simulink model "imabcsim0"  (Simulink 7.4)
settings: Solver=ode45  StartTime=0.0  StopTime=8  RelTol=1e-3
InitFcn:
  | imparamsim0
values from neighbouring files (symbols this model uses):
  Bm = 0.10    (= 0.1)    [IMabc2.m]    (also in imabcparam.m = 0.01; IMabcrun0.m = 0.01; IMabcrun1.m = 0.001; IMcur0.m = 1e-06)
  D = str2num(get(h,'string'))    [acttrcalc1.m]
  gam = 2*pi/3    (= 2.09439510239)    [IMabc2.m]    (also in IMabcf0.m; IMabcf1.m; imabcparam.m; IMabcrun0.m)
  J = 0.02    [imabcparam.m]    (also in IMabcrun0.m; IMabcrun1.m; imdefSIvec1.m = 0.03)
  Lm1 = 2/3*Lm    [IMabcf0.m]    (also in IMabcf1.m; imabcparam.m = 0.0564666666667; IMabcrun0.m = 0.0564666666667; IMabcrun1.m = 0.0564666666667)
  Lr = Lrl+Lm    (= 4.6)    [IMabc2.m]    (also in IMabcf0.m = Lrl+Lm1; IMabcf1.m = Lrl+Lm1; imabcparam.m = 0.0589666666667; IMcur0.m)
  Ls = Lsl+Lm    (= 4.6)    [IMabc2.m]    (also in IMabcf0.m = Lsl+Lm1; IMabcf1.m = Lsl+Lm1; imabcparam.m = 0.0589666666667; IMcur0.m)
  nsync = 120*freq0/p    (= 1800)    [imabcparam.m]
  p = cos(beta-alpha)    [abcRwdg.m]    (also in alternator.m = 0:pi/20:2*pi; altwdgs.m = 0:pi/20:2*pi; brushlessdcB.m = 0:pi/100:2*pi; brushlessdcnew.m = 0:pi/100:2*pi)
  Rr = input('Rotor resistance)[default = 2] =')    [Actac.m]    (also in im1phase.m = 0.3; im3d.m = eval(get(hRr,'String')); IMabc2.m = 0.02; imabcparam.m = 0.408)
  Rs = eval(get(hRs,'String'))    [im3d.m]    (also in IMabc2.m = 0.01; imabcparam.m = 0.531; IMabcrun0.m = 0.531; IMabcrun1.m = 0.531)
  Vm = Vll*sqrt(2/3)    [imabcparam.m]
  wo = 2*pi*freq0    [calc0.m]    (also in IMabc2.m = 376.991118431; imabcparam.m = 376.991118431; IMabcrun0.m = 376.991118431; IMabcrun1.m = 376.991118431)
undefined symbols (not defined in the file or in its folder): Row, TL1, TL2, vector

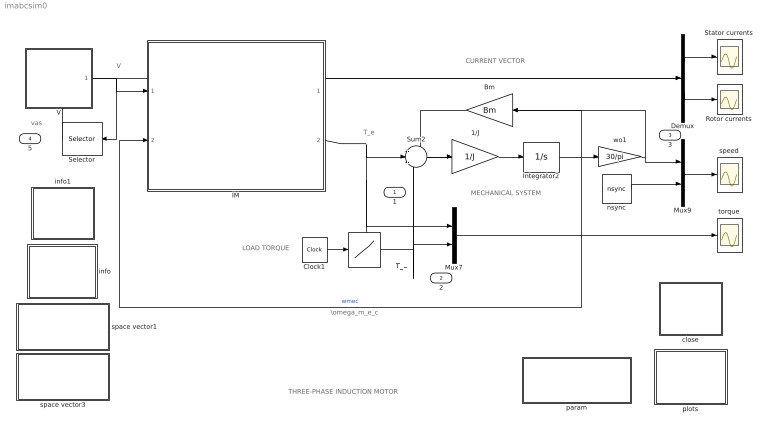
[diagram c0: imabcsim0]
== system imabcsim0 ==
  note: LOAD TORQUE
  note: T_L
  note: THREE-PHASE INDUCTION MOTOR
  note: T_e
  note: I
  note: MECHANICAL SYSTEM
  note: \omega_m_e_c
  note: CURRENT VECTOR
  note: V
  note: vas
  " " : Lookup  InputValues="[0 1.5 1.5  5 5 8]"  Table="[TL1 TL1  TL2 TL2 TL1 TL1]"  OutDataType=sfix(16)  OutScaling=2^0
  1/J : Gain  Gain=1/J  ParameterDataType=sfix(16)  ParameterScaling=2^0  OutDataType=sfix(16)  OutScaling=2^0
  Bm : Gain  Gain=Bm  ParameterDataType=sfix(16)  ParameterScaling=2^0  OutDataType=sfix(16)  OutScaling=2^0
  Clock1 : Clock
  Demux : Demux  Outputs=2
  IM : Subsystem
  Integrator2 : Integrator  InitialCondition=wo*2/p
  Mux7 : Mux  Inputs=2
  Mux9 : Mux  Inputs=2
  Rotor currents : Scope
  Selector : Selector  InputPortWidth=6  IndexOptions=Index vector (dialog)  Indices=1  OutputSizes=1
  Stator currents : Scope
  Sum2 : Sum  Inputs=-+-  OutDataType=sfix(16)  OutScaling=2^0
  V : Subsystem
  close : Subsystem
  info : Subsystem
  info1 : Subsystem
  nsync : Constant  Value=nsync  OutDataType=sfix(16)  OutScaling=2^0
  param : Subsystem
  plots : Subsystem
  space vector1 : Subsystem
  space vector3 : Subsystem
  speed : Scope
  torque : Scope
  wo1 : Gain  Gain=30/pi  ParameterDataType=sfix(16)  ParameterScaling=2^0  OutDataType=sfix(16)  OutScaling=2^0
  1 : Outport
  2 : Outport  Port=2
  3 : Outport  Port=3
  5 : Outport  Port=4
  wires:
  Demux/1 -> Stator currents/1
  Demux/2 -> Rotor currents/1
  V/1(V) -> IM/1(V), Selector/1
  IM/1(I) -> Demux/1
  Sum2/1 -> 1/J/1
  1/J/1 -> Integrator2/1
  Mux9/1 -> speed/1
  Integrator2/1 -> wo1/1, IM/2(wmec), Bm/1  "wmec"
  Mux7/1 -> torque/1
  " "/1 -> Mux7/2, Sum2/3, 2/1
  Clock1/1 -> " "/1
  IM/2(Te) -> Sum2/2, Mux7/1, 1/1
  nsync/1 -> Mux9/2
  Bm/1 -> Sum2/1
  wo1/1 -> Mux9/1, 3/1
  Selector/1 -> 5/1

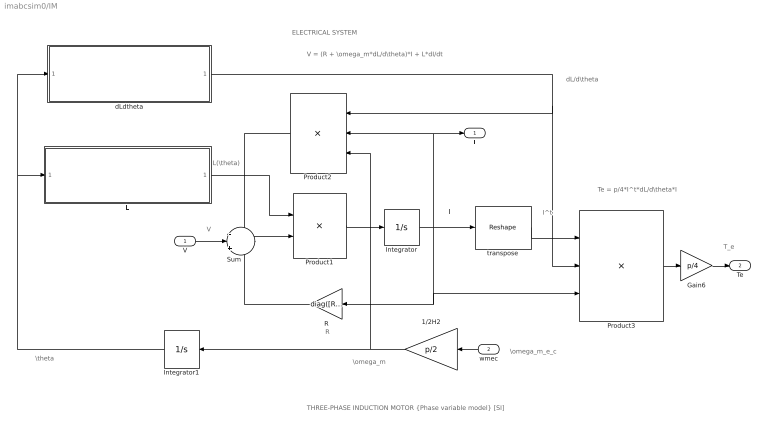
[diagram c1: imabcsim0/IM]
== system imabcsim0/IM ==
  note: I
  note: I^t
  note: ELECTRICAL SYSTEM
  note: V
  note: \omega_m
  note: \theta
  note: T_e
  note: dL/d\theta
  note: R
  note: V = (R + \omega_m*dL/d\theta)*I + L*dI/dt
  note: Te = p/4*I^t*dL/d\theta*I
  note: L(\theta)
  note: \omega_m_e_c
  note: THREE-PHASE INDUCTION MOTOR {Phase variable model} [SI]
  V : Inport  OutDataType=sfix(16)  OutScaling=2^0
  wmec : Inport  Port=2  OutDataType=sfix(16)  OutScaling=2^0
  1/2H2 : Gain  Gain=p/2  ParameterDataType=sfix(16)  ParameterScaling=2^0  OutDataType=sfix(16)  OutScaling=2^0
  Gain6 : Gain  Gain=p/4  ParameterDataType=sfix(16)  ParameterScaling=2^0  OutDataType=sfix(16)  OutScaling=2^0
  Integrator : Integrator  InitialCondition=[0 ;0 ;0; 0 ;0 ;0]
  Integrator1 : Integrator
  L : Subsystem
  Product1 : Product  Inputs=/*  Multiplication=Matrix(*)  OutDataType=sfix(16)  OutScaling=2^0
  Product2 : Product  Inputs=***  Multiplication=Matrix(*)  OutDataType=sfix(16)  OutScaling=2^0
  Product3 : Product  Inputs=3  Multiplication=Matrix(*)  OutDataType=sfix(16)  OutScaling=2^0
  R : Gain  Gain=diag([Rs Rs Rs Rr Rr Rr])  Multiplication=Matrix(K*u)  ParameterDataType=sfix(16)  ParameterScaling=2^0  OutDataType=sfix(16)  OutScaling=2^0
  Sum : Sum  Inputs=-|+|-  OutDataType=sfix(16)  OutScaling=2^0
  dLdtheta : Subsystem
  transpose : Reshape  OutputDimensionality=Row vector (2-D)  OutputDimensions=[1,6]
  I : Outport
  Te : Outport  Port=2
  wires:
  Product1/1 -> Integrator/1
  Integrator/1 -> Product3/3, R/1, transpose/1, Product2/2, I/1
  Sum/1 -> Product1/2
  R/1 -> Sum/3
  transpose/1 -> Product3/1
  Product2/1 -> Sum/1
  dLdtheta/1(dLdtheta) -> Product3/2, Product2/1
  Product3/1 -> Gain6/1
  1/2H2/1 -> Integrator1/1, Product2/3
  Integrator1/1 -> dLdtheta/1(theta1), L/1(theta)
  L/1(L) -> Product1/1
  V/1 -> Sum/2
  Gain6/1 -> Te/1
  wmec/1 -> 1/2H2/1

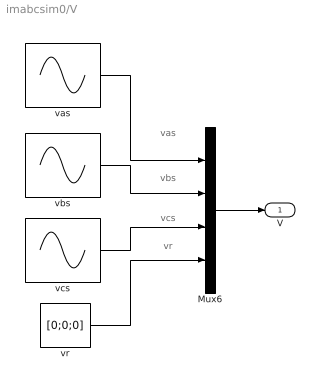
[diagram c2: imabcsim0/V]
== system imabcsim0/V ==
  note: vas
  note: vbs
  note: vcs
  note: vr
  Mux6 : Mux
  vas : Sin  Amplitude=Vm  Bias=0  Frequency=wo  Phase=pi/2  Samples=10  SampleTime=0
  vbs : Sin  Amplitude=Vm  Bias=0  Frequency=wo  Phase=pi/2-gam  Samples=10  SampleTime=0
  vcs : Sin  Amplitude=Vm  Bias=0  Frequency=wo  Phase=pi/2+gam  Samples=10  SampleTime=0
  vr : Constant  Value=[0;0;0]  VectorParams1D=off  OutDataType=sfix(16)  OutScaling=2^0
  V : Outport
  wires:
  Mux6/1 -> V/1
  vr/1 -> Mux6/4
  vcs/1 -> Mux6/3
  vbs/1 -> Mux6/2
  vas/1 -> Mux6/1

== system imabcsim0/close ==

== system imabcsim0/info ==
  note: The three-phase motor is running in steady state at a specified load when a pulsating torque load is applied. The machine dynamic equations are based on a matrix equivalent formulation in Simulink in which the state variables are the phase variables, namely the stator currents ias, ibs, ics and the rotor currents iar, ibr, icr; the rotor speed wm; and the angular displacement theta between stator as_axis and rotor ar_axis. The parameters describing the electromechanical system are expressed in SI units and may be modified by accessing a data file obtained by clicking the PARAMETERS block. The torque developed, the speed, and the stator current are observed on the scopes . The torque-speed dynamic characteristics can then be obtained after double clicking the PLOTS block. Steady-state currents are also plotted. To run the identical operation of this motor now formulated in a Matlab script file, run > or double click block. To run the identical operation in the space variable model using DQ, access the Simulink model file > or double click block.
  note: INDUCTION MOTOR RUNNING UNDER PULSED LOADS (Phase variable model) SI units

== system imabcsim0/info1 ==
  note: This demonstration illustrates the dynamics of a synchronous generator, initially at no load, following a three-phase short circuit at the terminals.
  note: Synchronous machine transients under shortcircuit

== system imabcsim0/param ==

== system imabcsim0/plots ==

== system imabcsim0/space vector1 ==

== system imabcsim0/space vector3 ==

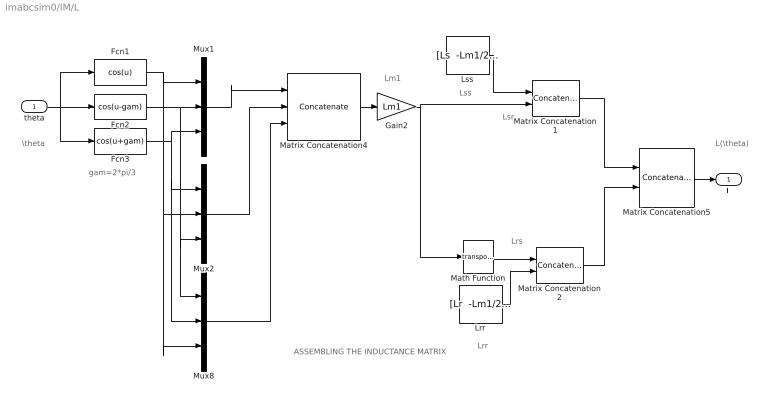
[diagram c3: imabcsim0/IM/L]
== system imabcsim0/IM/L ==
  note: ASSEMBLING THE INDUCTANCE MATRIX
  note: L(\theta)
  note: \theta
  note: gam=2*pi/3
  note: Lrr
  note: Lss
  note: Lsr
  note: Lrs
  note: Lm1
  theta : Inport  OutDataType=sfix(16)  OutScaling=2^0
  Fcn1 : Fcn  Expr=cos(u)
  Fcn2 : Fcn  Expr=cos(u-gam)
  Fcn3 : Fcn  Expr=cos(u+gam)
  Gain2 : Gain  Gain=Lm1  ParameterDataType=sfix(16)  ParameterScaling=2^0  OutDataType=sfix(16)  OutScaling=2^0
  Lrr : Constant  Value="[Lr  -Lm1/2  -Lm1/2; -Lm1/2  Lr -Lm1/2;-Lm1/2  -Lm1/2  Lr]"  VectorParams1D=off  OutDataType=sfix(16)  OutScaling=2^0
  Lss : Constant  Value="[Ls  -Lm1/2  -Lm1/2; -Lm1/2  Ls  -Lm1/2;-Lm1/2  -Lm1/2  Ls]"  VectorParams1D=off  OutDataType=sfix(16)  OutScaling=2^0
  Math Function : Math  Operator=transpose
  Matrix Concatenation1 : Concatenate  Mode=Multidimensional array  ConcatenateDimension=2
  Matrix Concatenation2 : Concatenate  Mode=Multidimensional array  ConcatenateDimension=2
  Matrix Concatenation4 : Concatenate  NumInputs=3  Mode=Multidimensional array  ConcatenateDimension=2
  Matrix Concatenation5 : Concatenate  Mode=Multidimensional array
  Mux1 : Mux  Inputs=3
  Mux2 : Mux  Inputs=3
  Mux8 : Mux  Inputs=3
  L : Outport
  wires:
  Matrix Concatenation5/1 -> L/1
  theta/1 -> Fcn3/1, Fcn1/1, Fcn2/1
  Math Function/1 -> Matrix Concatenation2/1
  Gain2/1 -> Matrix Concatenation1/2, Math Function/1
  Mux1/1 -> Matrix Concatenation4/1
  Matrix Concatenation4/1 -> Gain2/1
  Mux8/1 -> Matrix Concatenation4/3
  Mux2/1 -> Matrix Concatenation4/2
  Matrix Concatenation1/1 -> Matrix Concatenation5/1
  Matrix Concatenation2/1 -> Matrix Concatenation5/2
  Lss/1 -> Matrix Concatenation1/1
  Lrr/1 -> Matrix Concatenation2/2
  Fcn3/1 -> Mux1/3, Mux2/1, Mux8/2
  Fcn2/1 -> Mux1/2, Mux2/3, Mux8/1
  Fcn1/1 -> Mux8/3, Mux2/2, Mux1/1

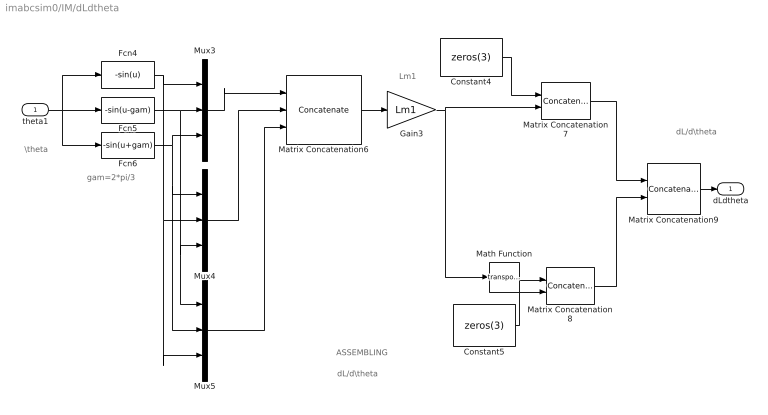
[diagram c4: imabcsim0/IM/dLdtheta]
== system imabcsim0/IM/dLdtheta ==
  note: dL/d\theta
  note: \theta
  note: gam=2*pi/3
  note: Lm1
  note: ASSEMBLING
  note: dL/d\theta
  theta1 : Inport  OutDataType=sfix(16)  OutScaling=2^0
  Constant4 : Constant  Value=zeros(3)  VectorParams1D=off  OutDataType=sfix(16)  OutScaling=2^0
  Constant5 : Constant  Value=zeros(3)  VectorParams1D=off  OutDataType=sfix(16)  OutScaling=2^0
  Fcn4 : Fcn  Expr=-sin(u)
  Fcn5 : Fcn  Expr=-sin(u-gam)
  Fcn6 : Fcn  Expr=-sin(u+gam)
  Gain3 : Gain  Gain=Lm1  ParameterDataType=sfix(16)  ParameterScaling=2^0  OutDataType=sfix(16)  OutScaling=2^0
  Math Function : Math  Operator=transpose
  Matrix Concatenation6 : Concatenate  NumInputs=3  Mode=Multidimensional array  ConcatenateDimension=2
  Matrix Concatenation7 : Concatenate  Mode=Multidimensional array  ConcatenateDimension=2
  Matrix Concatenation8 : Concatenate  Mode=Multidimensional array  ConcatenateDimension=2
  Matrix Concatenation9 : Concatenate  Mode=Multidimensional array
  Mux3 : Mux  Inputs=3
  Mux4 : Mux  Inputs=3
  Mux5 : Mux  Inputs=3
  dLdtheta : Outport
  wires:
  Matrix Concatenation9/1 -> dLdtheta/1
  theta1/1 -> Fcn5/1, Fcn4/1, Fcn6/1
  Gain3/1 -> Matrix Concatenation7/2, Math Function/1
  Mux4/1 -> Matrix Concatenation6/2
  Mux3/1 -> Matrix Concatenation6/1
  Matrix Concatenation6/1 -> Gain3/1
  Mux5/1 -> Matrix Concatenation6/3
  Matrix Concatenation7/1 -> Matrix Concatenation9/1
  Matrix Concatenation8/1 -> Matrix Concatenation9/2
  Constant4/1 -> Matrix Concatenation7/1
  Constant5/1 -> Matrix Concatenation8/2
  Fcn6/1 -> Mux3/3, Mux4/1, Mux5/2
  Fcn5/1 -> Mux3/2, Mux4/3, Mux5/1
  Fcn4/1 -> Mux3/1, Mux4/2, Mux5/3
  Math Function/1 -> Matrix Concatenation8/1
